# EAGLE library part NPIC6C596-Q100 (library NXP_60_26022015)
NPIC6C596-Q100 The NPIC6C596-Q100 is an 8-bit serial-in/serial or parallel-out shift register with a storage register and open-drain outputs. Both the shift and storage register have separate clocks. The device features a serial input (DS) and a serial output (Q7S) to enable cascading and an asynchronous reset MR input. A LOW on MR resets both the shift register and storage register. Data is shifted on the LOW-to-HIGH transitions of the SHCP input. The data in the shift register is transferred to the storage register on a LOW-to-HIGH transition of the STCP input. If both clocks are connected together, the shift register is always one clock pulse ahead of the storage register. To provide additional hold time in cascaded applications, the serial output QS7 is clocked out on the falling edge of SHCP. Data in the storage register drives the gate of the output extended-drain NMOS (EDNMOS) transistor whenever the output enable input (OE) is LOW. A HIGH on OE causes the outputs to assume a high-impedance OFF-state. Operation of the OE input does not affect the state of the registers. The open-drain outputs are 33 V/100 mA continuous current extended-drain NMOS transistors designed for use in systems that require moderate load power such as LEDs. Integrated voltage clamps in the outputs provide protection against inductive transients making the device suitable for power driver applications such as relays, solenoids and other low-current or medium-voltage loads. This product has been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
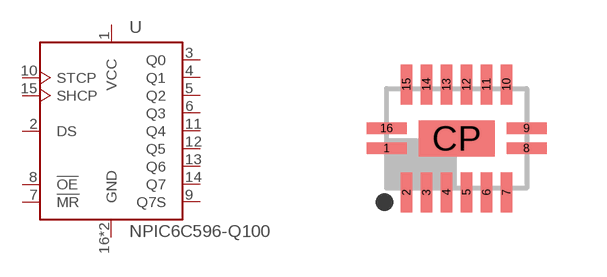
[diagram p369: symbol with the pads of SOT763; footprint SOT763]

Designator prefix U

## NPIC6C596-Q100  [SOT763]
1  VCC
2  DS  in
3  Q0  oc
4  Q1  oc
5  Q2  oc
6  Q3  oc
7  !MR  in
8  !OE  in
9  Q7S  out
10  STCP  in
11  Q4  oc
12  Q5  oc
13  Q6  oc
14  Q7  oc
15  SHCP  in
16  GND
CP  GND

## Footprint SOT763 (pad centres in mm)
SOT763 DHVQFN16: plastic dual in-line compatible thermal enhanced very thin quad flat package; no leads; 16 terminals; body 2.5 x 3.5 x 0.85 mm JEDEC: MO-241 IEC: -- JEITA: --
smd 1 x 0.29: 1 -1.75,-0.25; 8 1.75,-0.25; 9 1.75,0.25; 16 -1.75,0.25
smd 0.29 x 1: 2 -1.25,-1.35; 3 -0.75,-1.35; 4 -0.25,-1.35; 5 0.25,-1.35; 6 0.75,-1.35; 7 1.25,-1.35; 10 1.25,1.35; 11 0.75,1.35; 12 0.25,1.35; 13 -0.25,1.35; 14 -0.75,1.35; 15 -1.25,1.35
smd 1.9 x 0.9: CP 0,0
